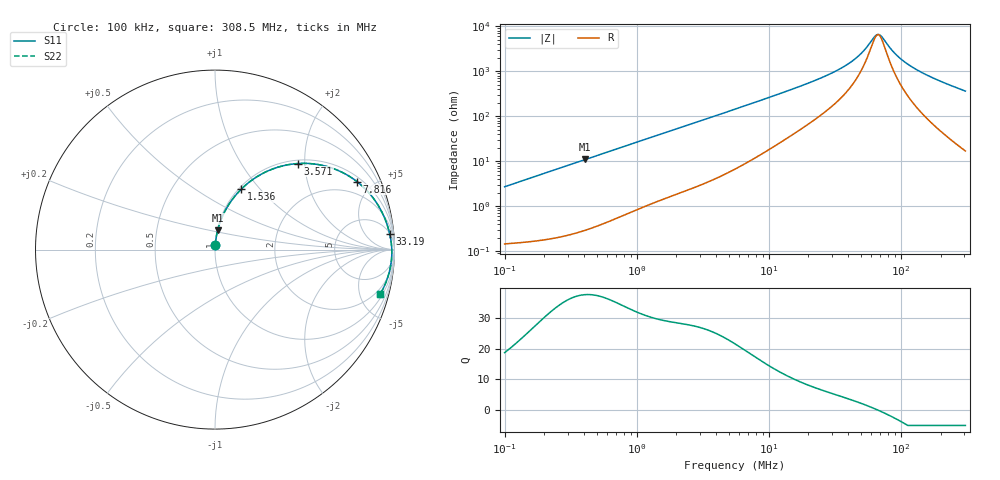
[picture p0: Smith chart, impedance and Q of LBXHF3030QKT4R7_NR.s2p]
! LBXHF3030QKT4R7_NR  S-PARAMETER MODEL  ( General Type )
! Model Generated by TAIYO YUDEN Corporation (http://www.ty-top.com)
! Version 1.0
! TAIYO YUDEN Control No. 210113NI43SB-FBB
! Copyright(c) 2021 TAIYO YUDEN CO.,LTD. All Rights Reserved.
! Product Description (link to TY-COMPAS)
! https://ds.yuden.co.jp/TYCOMPAS/or/detail?pn=LBXHF3030QKT4R7MNR&u=M
! Products Name : Inductors
! Characteristics :
!  Inductance : 4.7 uH , SRF(min) : 40 MHz , DC Resistance(max) : 0.12 Ohm
!  Rated Current : Saturation :1000 mA , Temp Rise : 1000 mA
!  Case Size : 3.0 x 3.0 / 0.118 x 0.118 [mm/inch] , Thickness : 1.5 / 0.059 [mm/inch]
!  (Conditions: Temperature = 25 degC , DC Bias Current/Voltage = 0A / 0V)
! External Node Assignments :
!  1  o---GGG---o  2
! GND o---------o GND
! Frequency Range : 0.1MHz  -  308.54851MHz  [ 402 STEP ]
# MHz S RI R 50
! Freq[MHz].  S11 Real  S11 Imag  S21 Real  S21 Imag  S12 Real  S12 Imag  S22 Real  S22 Imag
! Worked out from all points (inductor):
!   401 points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, 100 kHz to 308.5 MHz, reference 50 ohm
!   read as one part in series: L = 4.28 uH near 104.1 kHz
!   highest Q = 37.6 at 408 kHz (marker M1), where L = 4.25 uH
!   self-resonance near 67.04 MHz
!   S11 on the Smith chart (normalised r, x): 100 kHz: 1.00, +0.05; 1.536 MHz: 1.03, +0.80; 3.571 MHz: 1.07, +1.85; 7.816 MHz: 1.23, +4.05; 33.19 MHz: 5, +21; 308.5 MHz: 1.34, -7.25
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0.1  0.00216 0.0268  0.9978 -0.0268  0.9978 -0.0268  0.00216 0.0268
0.384115  0.0131 0.101  0.9869 -0.101  0.9869 -0.101  0.0131 0.101
0.407973  0.0145 0.107  0.9855 -0.107  0.9855 -0.107  0.0145 0.107
0.857816  0.0549 0.2132  0.9451 -0.2132  0.9451 -0.2132  0.0549 0.2132
1.475446  0.1384 0.3288  0.8616 -0.3288  0.8616 -0.3288  0.1384 0.3288
1.535925  0.1476 0.3381  0.8524 -0.3381  0.8524 -0.3381  0.1476 0.3381
2.295283  0.2699 0.4264  0.7301 -0.4264  0.7301 -0.4264  0.2699 0.4264
3.570664  0.462 0.4796  0.538 -0.4796  0.538 -0.4796  0.462 0.4796
5.667415  0.6747 0.4457  0.3253 -0.4457  0.3253 -0.4457  0.6747 0.4457
7.815522  0.7909 0.3789  0.2091 -0.3789  0.2091 -0.3789  0.7909 0.3789
12.15824  0.8925 0.272  0.1075 -0.272  0.1075 -0.272  0.8925 0.272
21.33651  0.9528 0.1566  0.0472 -0.1566  0.0472 -0.1566  0.9528 0.1566
33.19221  0.9733 0.0882  0.0267 -0.0882  0.0267 -0.0882  0.9733 0.0882
40.57601  0.9786 0.0615  0.0214 -0.0615  0.0214 -0.0615  0.9786 0.0615
47.64921  0.9817 0.0414  0.0183 -0.0414  0.0183 -0.0414  0.9817 0.0414
65.70958  0.985 0.00262  0.015 -0.00262  0.015 -0.00262  0.985 0.00262
71.20687  0.9853 -0.00705  0.0147 0.00705  0.0147 0.00705  0.9853 -0.00705
81.95682  0.9852 -0.0242  0.0148 0.0242  0.0148 0.0242  0.9852 -0.0242
100.1886  0.9838 -0.0498  0.0162 0.0498  0.0162 0.0498  0.9838 -0.0498
130.0832  0.9793 -0.086  0.0207 0.086  0.0207 0.086  0.9793 -0.086
190.5303  0.9643 -0.1485  0.0357 0.1485  0.0357 0.1485  0.9643 -0.1485
308.5485  0.9195 -0.2499  0.0805 0.2499  0.0805 0.2499  0.9195 -0.2499
